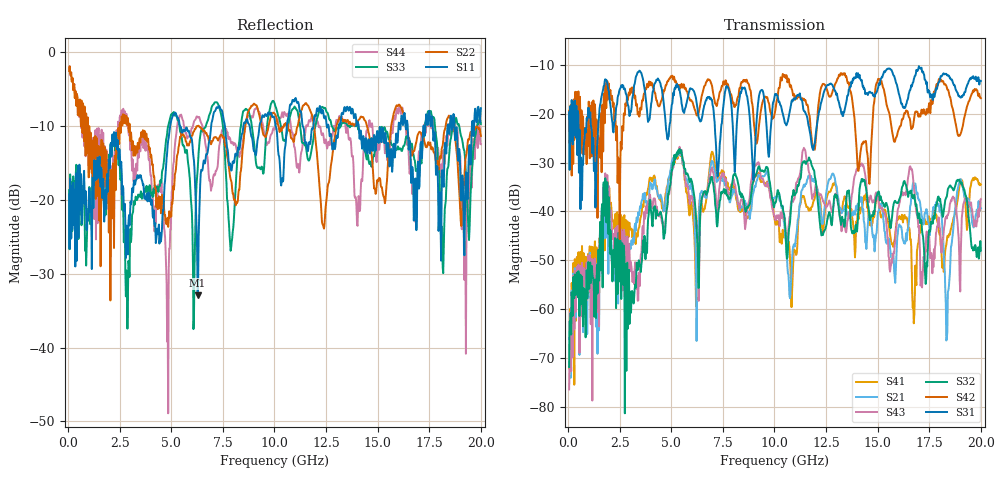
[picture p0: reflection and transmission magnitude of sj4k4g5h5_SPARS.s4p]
! FILE: E:\users\goganessyan\GBX_Backplane\FR408_backplane\1m_INBOUND_NEXT\sj4k4g5h5_SPARS.s4p
# MHZ S RI R 50.00
! FREQ  S11  S12  S13  S14
!  S21  S22  S23  S24
!  S31  S32  S33  S34
!  S41  S42  S43  S44
!  REAL  IMAG  REAL  IMAG  REAL  IMAG  REAL  IMAG
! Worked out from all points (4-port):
!   799 points, 50 MHz to 20 GHz, reference 50 ohm
!   strongest paths, dB at 50 MHz, 5.025 GHz, 10.03 GHz, 15.03 GHz, 20 GHz:
!     S31: -19.7, -18.1, -16.0, -14.6, -13.3
!     S42: -19.4, -12.6, -19.6, -12.9, -16.8
!     S32: -71.8, -31.5, -38.2, -36.1, -48.0
!     S43: -76.4, -32.5, -41.5, -37.6, -37.5
!     S21: -66.1, -29.8, -37.1, -40.0, -39.4
!     S41: -72.0, -31.0, -42.1, -36.9, -34.5
!   lowest |S11| = -32.9 dB at 6.275 GHz (marker M1), VSWR 1.05, Z = 51.7 - j1.52 ohm
!   |S11| at or under -10 dB: start of sweep to 4.943 GHz; 5.423 GHz to 6.931 GHz (1.508 GHz wide, 24.4 % of centre); 14.08 GHz to 16.01 GHz (1.931 GHz wide, 12.8 % of centre)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
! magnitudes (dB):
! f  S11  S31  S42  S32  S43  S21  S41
! 50 MHz  -19.3  -19.7  -19.4  -71.8  -76.4  -66.1  -72.0
! 1.85 GHz  -21.2  -13.1  -18.9  -42.2  -39.7  -45.3  -40.5
! 2.825 GHz  -24.9  -16.1  -18.4  -72.6  -55.8  -46.8  -45.3
! 4.8 GHz  -13.6  -25.0  -13.5  -39.1  -39.0  -35.5  -34.8
! 6.275 GHz  -32.9  -19.1  -20.2  -47.4  -46.0  -50.1  -46.8
! 16.75 GHz  -22.8  -13.0  -21.5  -36.9  -34.9  -34.8  -62.9
! 20 GHz  -7.6  -13.3  -16.8  -48.0  -37.5  -39.4  -34.5
